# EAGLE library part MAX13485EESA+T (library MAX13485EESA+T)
MAXIM INTEGRATED PRODUCTS - MAX13485EESA+T - Transceiver RS422, RS485, 4.75V-5.25V supply, 1 Driver, NSOIC-8 Source: Datasheet
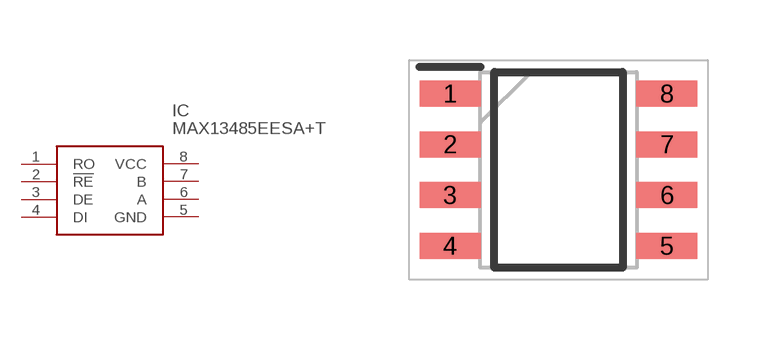
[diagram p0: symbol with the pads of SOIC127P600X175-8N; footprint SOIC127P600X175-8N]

Designator prefix IC

## MAX13485EESA+T (Arrow_Part_Number: MAX13485EESA+T; Arrow_Price-Stock: https://www.arrow.com/en/products/max13485eesat/maxim-integrated?region=nac; Description: MAXIM INTEGRATED PRODUCTS - MAX13485EESA+T - Transceiver RS422, RS485, 4.75V-5.25V supply, 1 Driver, NSOIC-8; Height: 1.75mm; Manufacturer_Name: Maxim Integrated; Manufacturer_Part_Number: MAX13485EESA+T; Mouser_Part_Number: 700-MAX13485EESAT; Mouser_Price-Stock: https://www.mouser.co.uk/ProductDetail/Maxim-Integrated/MAX13485EESA%2bT?qs=CDqwynd4ZNrGM4Km3K5uAA%3D%3D)  [SOIC127P600X175-8N]
1  RO
2  !RE
3  DE
4  DI
5  GND
6  A
7  B
8  VCC

## Footprint SOIC127P600X175-8N (pad centres in mm)
S8+2
smd 1.525 x 0.65: 1 -2.712,1.905; 2 -2.712,0.635; 3 -2.712,-0.635; 4 -2.712,-1.905; 5 2.712,-1.905; 6 2.712,-0.635; 7 2.712,0.635; 8 2.712,1.905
